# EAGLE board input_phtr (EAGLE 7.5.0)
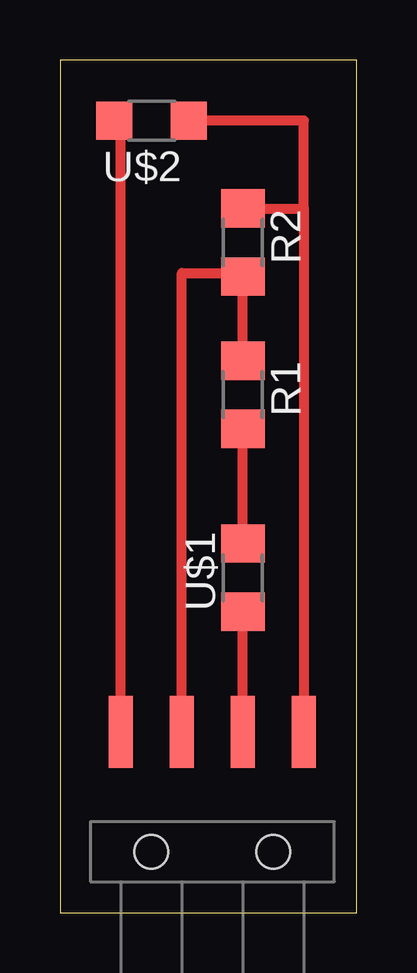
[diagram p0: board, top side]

Size 12.37 x 35.55 mm. Coordinates in mm from the lower left corner, seen from the top.
Outline: 0,0 12.37,0 12.37,35.55 0,35.55 0,0
Copper layers (1*16): Top 0.035mm / dielectric 1.5mm / Bottom 0.035mm
Design rules "default": minimum track width 10mil, minimum drill 24mil, track to track 8mil, track to pad 8mil, pad to pad 8mil, via to via 8mil, smd to smd 8mil, copper to edge 40mil, drill to drill 8mil, minimum pad ring 10mil, minimum via ring 8mil, stop-mask expansion 4mil, vias tented up to drill 0mil, thermal gap 10mil

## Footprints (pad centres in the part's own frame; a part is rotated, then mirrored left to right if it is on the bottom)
1X04-SMD = smd 1 x 3: 1 -3.81,5; 2 -1.27,5; 3 1.27,5; 4 3.81,5 | hole 1.4: -2.54,0; 2.54,0
1206 = smd 1.6 x 1.803: 1 -1.422,0; 2 1.422,0
OP1206 = smd 1.5 x 1.6: COLLECTOR -1.55,0; EMITTER 1.55,0

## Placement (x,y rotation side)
JP1  [1X04-SMD]  6.35,2.54 0 top
R1  499  [1206]  7.62,21.59 270 top
R2  10K  [1206]  7.62,27.94 270 top
U$1  [1206]  7.62,13.97 90 top
U$2  PHOTOTRANSISTOR-NPN1206  [OP1206]  3.81,33.02 180 top

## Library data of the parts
JP1 = 01_SparkFun
R1 R2 U$1 = 01_FAB_Hello
U$2 = 01_fab

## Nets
GND: JP1.2 R1.1 R2.2
IN: JP1.4 R2.1 U$2.COLLECTOR
N$1: R1.2 U$1.2
OUT: JP1.3 U$1.1
VCC: JP1.1 U$2.EMITTER

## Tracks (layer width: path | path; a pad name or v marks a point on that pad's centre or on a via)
GND
  Top 0.406: JP1.2 5.08,26.67 7.47,26.67 R2.2 R1.1
IN
  Top 0.406: R2.1 10.16,29.36 | 10.16,29.36 JP1.4 | 10.16,29.36 10.16,33.02 U$2.COLLECTOR
N$1
  Top 0.406: U$1.2 R1.2
OUT
  Top 0.406: JP1.3 U$1.1
VCC
  Top 0.406: JP1.1 2.54,32.74 U$2.EMITTER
